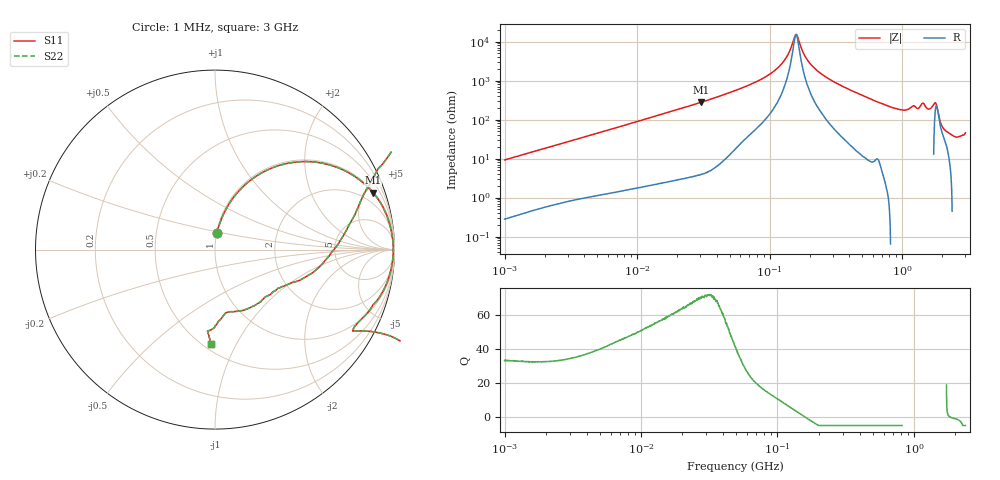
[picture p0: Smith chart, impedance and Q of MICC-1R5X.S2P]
!s-Parameter Generated by FASTRON Sdn. Bhd.
!FASTRON P/N : MICC-1R5X
!Keysight Technologies,E4991B,MY54100416,A.01.15
!Date: Fri Aug 28 09:23:59 2026
!Version  : Rev00 Fri Aug 28 09:23:59 2026
!Data & Calibration Information:
!PortZ  Port1:50+j0  Port2:50+j0
!When reading, reference impedance value at option line is always used.
!Remarks : This data is being provided solely for informational purposes.
!Freq	S11	S21	S12	S22
# Hz S dB R 50
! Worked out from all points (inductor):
!   1601 points, 1 MHz to 3 GHz, reference 50 ohm
!   read as one part in series: L = 1.46 uH near 1.041 MHz
!   highest Q = 71.3 at 30.2 MHz (marker M1), where L = 1.46 uH
!   self-resonance near 158.2 MHz
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1000000  -20.76 83.0  -0.06 -5.3  -0.06 -5.3  -20.76 83.0
3804036  -9.88 69.7  -0.55 -18.7  -0.55 -18.7  -9.88 69.7
1.447069e7  -2.12 37.4  -4.32 -51.6  -4.32 -51.6  -2.12 37.4
3.019602e7  -0.57 19.8  -9.40 -69.4  -9.40 -69.4  -0.57 19.8
5.477226e7  -0.19 10.2  -15.06 -78.1  -15.06 -78.1  -0.19 10.2
1.131553e8  -0.07 2.8  -26.14 -79.8  -26.14 -79.8  -0.07 2.8
1.341416e8  -0.06 1.4  -32.12 -73.8  -32.12 -73.8  -0.06 1.4
1.574367e8  -0.06 0.1  -43.59 -8.1  -43.59 -8.1  -0.06 0.1
1.847772e8  -0.06 -1.3  -32.66 72.3  -32.66 72.3  -0.06 -1.3
2.083556e8  -0.07 -2.3  -27.77 78.3  -27.77 78.3  -0.07 -2.3
3.268837e8  -0.12 -6.9  -18.43 80.0  -18.43 80.0  -0.12 -6.9
7.925923e8  -0.83 -24.5  -7.65 65.3  -7.65 65.3  -0.83 -24.5
1.091779e9  -0.86 -30.1  -5.97 64.5  -5.97 64.5  -0.86 -30.1
1.327057e9  2.58 -29.9  -3.20 103.9  -3.20 103.9  2.58 -29.9
1.402151e9  3.32 -17.3  -4.58 132.5  -4.58 132.5  3.32 -17.3
1.488926e9  4.77 10.4  -2.28 -155.9  -2.28 -155.9  4.77 10.4
1.54974e9  4.42 25.4  -1.19 -125.2  -1.19 -125.2  4.42 25.4
1.604986e9  3.09 30.9  -2.30 -107.0  -2.30 -107.0  3.09 30.9
1.791767e9  -2.38 10.5  -10.82 -28.7  -10.82 -28.7  -2.38 10.5
1.990301e9  -7.08 -26.6  -3.93 18.1  -3.93 18.1  -7.08 -26.6
2.556106e9  -8.99 -78.6  -0.06 20.5  -0.06 20.5  -8.99 -78.6
3e9  -5.56 -92.5  1.22 27.2  1.22 27.2  -5.56 -92.5
